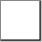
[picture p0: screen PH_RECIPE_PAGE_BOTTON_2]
VISUALIZATION PH_RECIPE_PAGE_BOTTON_2  // 42x42
VAR_IN_OUT
	RECIPE_CTRL_V2 : None;
END_VAR
    Rectangle (0,0 40x40)
        tap RECIPE_CTRL_V2.sCmd.bJumpBottom
    Polyline (35,30), colour toggle: (RECIPE_CTRL_V2.sCmd.bJumpBottom) <> 0
        tap RECIPE_CTRL_V2.sCmd.bJumpBottom
    Polygon (20,20), colour toggle: (RECIPE_CTRL_V2.sCmd.bJumpBottom) <> 0
        tap RECIPE_CTRL_V2.sCmd.bJumpBottom
    Polygon (20,30), colour toggle: (RECIPE_CTRL_V2.sCmd.bJumpBottom) <> 0
        tap RECIPE_CTRL_V2.sCmd.bJumpBottom
END_VISUALIZATION
